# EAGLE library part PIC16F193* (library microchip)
Flash-Based, 8-Bit CMOS Microcontrollers wtih LCD Driver and nanoWatt XLP Technology Auto generated by make-symbol-device-package-bsdl.ulp Rev. 33 Source: http://ww1.microchip.com/downloads/en/DeviceDoc/41364D.pdf
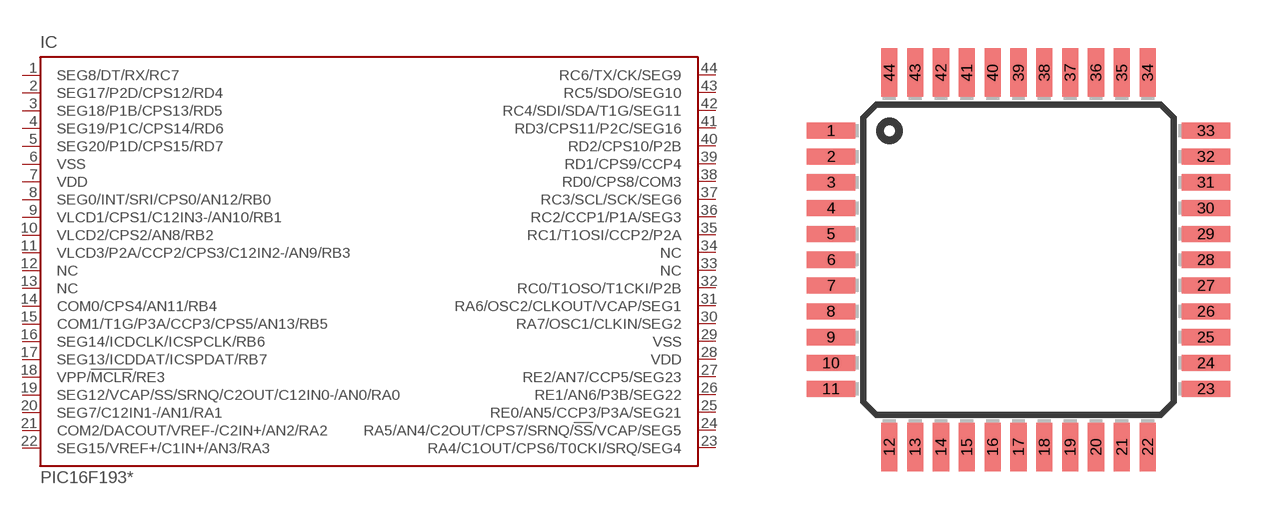
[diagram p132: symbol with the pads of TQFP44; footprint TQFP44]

Designator prefix IC

## PIC16F1934PT (MPN: PIC16F1934-I/PT; OC_FARNELL: 1755818; OC_NEWARK: 34R4514), PIC16F1937PT (MPN: PIC16F1937-I/PT; OC_FARNELL: 1755826; OC_NEWARK: 34R4521), PIC16F1939PT (MPN: PIC16F1939-I/PT; OC_FARNELL: 1755834; OC_NEWARK: 08R1959)  [TQFP44]
1  SEG8/DT/RX/RC7
2  SEG17/P2D/CPS12/RD4
3  SEG18/P1B/CPS13/RD5
4  SEG19/P1C/CPS14/RD6
5  SEG20/P1D/CPS15/RD7
6  VSS  pwr
7  VDD  pwr
8  SEG0/INT/SRI/CPS0/AN12/RB0
9  VLCD1/CPS1/C12IN3-/AN10/RB1
10  VLCD2/CPS2/AN8/RB2
11  VLCD3/P2A/CCP2/CPS3/C12IN2-/AN9/RB3
12  NC  nc
13  NC  nc
14  COM0/CPS4/AN11/RB4
15  COM1/T1G/P3A/CCP3/CPS5/AN13/RB5
16  SEG14/ICDCLK/ICSPCLK/RB6
17  SEG13/ICDDAT/ICSPDAT/RB7
18  VPP/!MCLR!/RE3  in
19  SEG12/VCAP/SS/SRNQ/C2OUT/C12IN0-/AN0/RA0
20  SEG7/C12IN1-/AN1/RA1
21  COM2/DACOUT/VREF-/C2IN+/AN2/RA2
22  SEG15/VREF+/C1IN+/AN3/RA3
23  RA4/C1OUT/CPS6/T0CKI/SRQ/SEG4
24  RA5/AN4/C2OUT/CPS7/SRNQ/!SS!/VCAP/SEG5
25  RE0/AN5/CCP3/P3A/SEG21
26  RE1/AN6/P3B/SEG22
27  RE2/AN7/CCP5/SEG23
28  VDD  pwr
29  VSS  pwr
30  RA7/OSC1/CLKIN/SEG2
31  RA6/OSC2/CLKOUT/VCAP/SEG1
32  RC0/T1OSO/T1CKI/P2B
33  NC  nc
34  NC  nc
35  RC1/T1OSI/CCP2/P2A
36  RC2/CCP1/P1A/SEG3
37  RC3/SCL/SCK/SEG6
38  RD0/CPS8/COM3
39  RD1/CPS9/CCP4
40  RD2/CPS10/P2B
41  RD3/CPS11/P2C/SEG16
42  RC4/SDI/SDA/T1G/SEG11
43  RC5/SDO/SEG10
44  RC6/TX/CK/SEG9

## Footprint TQFP44 (pad centres in mm)
Thin Quad Flat Pack package type TQ
smd 1.5 x 0.5: 1 -5.8,4; 2 -5.8,3.2; 3 -5.8,2.4; 4 -5.8,1.6; 5 -5.8,0.8; 6 -5.8,0; 7 -5.8,-0.8; 8 -5.8,-1.6; 9 -5.8,-2.4; 10 -5.8,-3.2; 11 -5.8,-4; 23 5.8,-4; 24 5.8,-3.2; 25 5.8,-2.4; 26 5.8,-1.6; 27 5.8,-0.8; 28 5.8,0; 29 5.8,0.8; 30 5.8,1.6; 31 5.8,2.4; 32 5.8,3.2; 33 5.8,4
smd 0.5 x 1.5: 12 -4,-5.8; 13 -3.2,-5.8; 14 -2.4,-5.8; 15 -1.6,-5.8; 16 -0.8,-5.8; 17 0,-5.8; 18 0.8,-5.8; 19 1.6,-5.8; 20 2.4,-5.8; 21 3.2,-5.8; 22 4,-5.8; 34 4,5.8; 35 3.2,5.8; 36 2.4,5.8; 37 1.6,5.8; 38 0.8,5.8; 39 0,5.8; 40 -0.8,5.8; 41 -1.6,5.8; 42 -2.4,5.8; 43 -3.2,5.8; 44 -4,5.8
